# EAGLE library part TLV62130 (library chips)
High Efficient 3A switching step-down regulator. 1V-5V out, 4V-17V in.
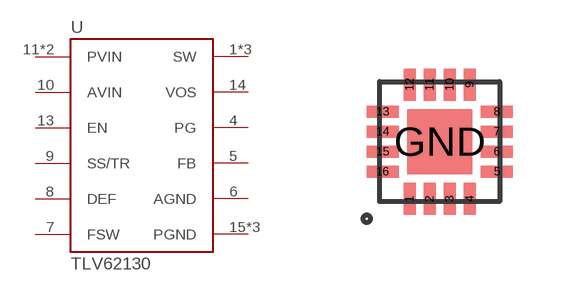
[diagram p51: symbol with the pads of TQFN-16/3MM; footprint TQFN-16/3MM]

Designator prefix U

## TLV62130 (DIGIKEY: 296-35978-1-ND; MANUFACTURER: Texas Instruments; MPN: TLV62130RGTR)  [TQFN-16/3MM]
1  SW
2  SW
3  SW
4  PG
5  FB
6  AGND
7  FSW
8  DEF
9  SS/TR
10  AVIN
11  PVIN
12  PVIN
13  EN
14  VOS
15  PGND
16  PGND
GND  PGND

## Footprint TQFN-16/3MM (pad centres in mm)
smd 0.3 x 0.8: 1 -0.75,-1.43; 2 -0.25,-1.43; 3 0.25,-1.43; 4 0.75,-1.43; 9 0.75,1.43; 10 0.25,1.43; 11 -0.25,1.43; 12 -0.75,1.43
smd 0.8 x 0.3: 5 1.43,-0.75; 6 1.43,-0.25; 7 1.43,0.25; 8 1.43,0.75; 13 -1.43,0.75; 14 -1.43,0.25; 15 -1.43,-0.25; 16 -1.43,-0.75
smd 1.63 x 1.63: GND 0,0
